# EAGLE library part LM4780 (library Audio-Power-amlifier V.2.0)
The LM4780 is an stereo audio amplifier capable of typically delivering 60W per channel of continuous average output power into an 8Ω load with less than 0.5% THD+N from 20Hz - 20kHz. The LM4780 is fully protected utilizing National's Self Peak Instantaneous Temperature (°Ke) (SPiKeTM) protection circuitry. SPiKe provides a dynamically optimized Safe Operating Area (SOA). SPiKe protection completely safeguards the LM4780's outputs against over-voltage, under-voltage, overloads, shorts to the supplies or GND, thermal runaway and instantaneous temperature peaks. The advanced protection features of the LM4780 places it in a class above discrete and hybrid amplifiers. Each amplifier of the LM4780 has an independent smooth transition fade-in/out mute. The LM4780 can easily be configured for bridge or parallel operation for 120W mono solutions.
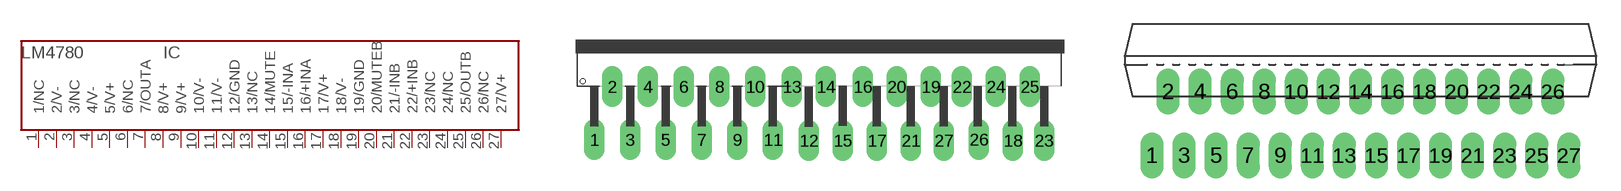
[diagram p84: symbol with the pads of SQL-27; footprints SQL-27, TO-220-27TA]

Designator prefix IC

## LM4780  [SQL-27]
1  1/NC  nc
2  2/V-  pwr
3  3/NC  nc
4  4/V-  pwr
5  5/V+  pwr
6  6/NC  nc
7  7/OUTA  out
8  8/V+  pwr
9  9/V+  pwr
10  10/V-  pwr
11  11/V-  pwr
12  12/GND  pwr
13  13/NC  nc
14  14/MUTE  in
15  15/-INA  in
16  16/+INA  in
17  17/V+  pwr
18  18/V-  pwr
19  19/GND  pwr
20  20/MUTEB  in
21  21/-INB  in
22  22/+INB  in
23  23/NC  nc
24  24/NC  nc
25  25/OUTB  out
26  26/NC  nc
27  27/V+  pwr

## LM4780LM4780BD  [TO-220-27TA]
Pads as for SQL-27

## Footprint SQL-27 (pad centres in mm)
drill 1.3 long: 1 -7.239,1.905; 2 -5.537,6.96; 3 -3.835,1.905; 4 -2.134,6.96; 5 -0.432,1.905; 6 1.27,6.96; 7 2.972,1.905; 8 4.674,6.96; 9 6.375,1.905; 10 8.077,6.96; 11 9.779,1.905; 12 13.207,1.83; 13 11.587,6.96; 14 14.827,6.96; 15 16.447,1.83; 16 18.337,6.96; 17 19.687,1.83; 18 32.647,1.83; 19 24.817,6.96; 20 21.577,6.96; 21 22.927,1.83; 22 27.787,6.96; 23 35.617,1.83; 24 31.027,6.96; 25 34.267,6.96; 26 29.407,1.93; 27 26.067,1.83

## Footprint TO-220-27TA (pad centres in mm)
TO-220_MKT-TA27A , MOLDED (inch. 1,150x0,618x0,177 - body_0,040 pitch )
drill 0.5 pad 1.422 long: 1 -13.007,-3.988; 2 -12.009,0; 3 -11.008,-3.988; 4 -10.008,0; 5 -9.007,-3.988; 6 -8.006,0; 7 -7.005,-3.988; 8 -6.002,0; 9 -5.004,-3.988; 10 -4.003,0; 11 -3.002,-3.988; 12 -1.999,0; 13 -1.001,-3.99; 14 0,0; 15 1.001,-3.988; 16 2.002,0; 17 3.002,-3.988; 18 4.003,0; 19 5.004,-3.988; 20 6.007,0; 21 7.005,-3.988; 22 8.006,0; 23 9.009,-3.988; 24 10.008,0; 25 11.008,-3.988; 26 12.009,0; 27 13.01,-3.988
